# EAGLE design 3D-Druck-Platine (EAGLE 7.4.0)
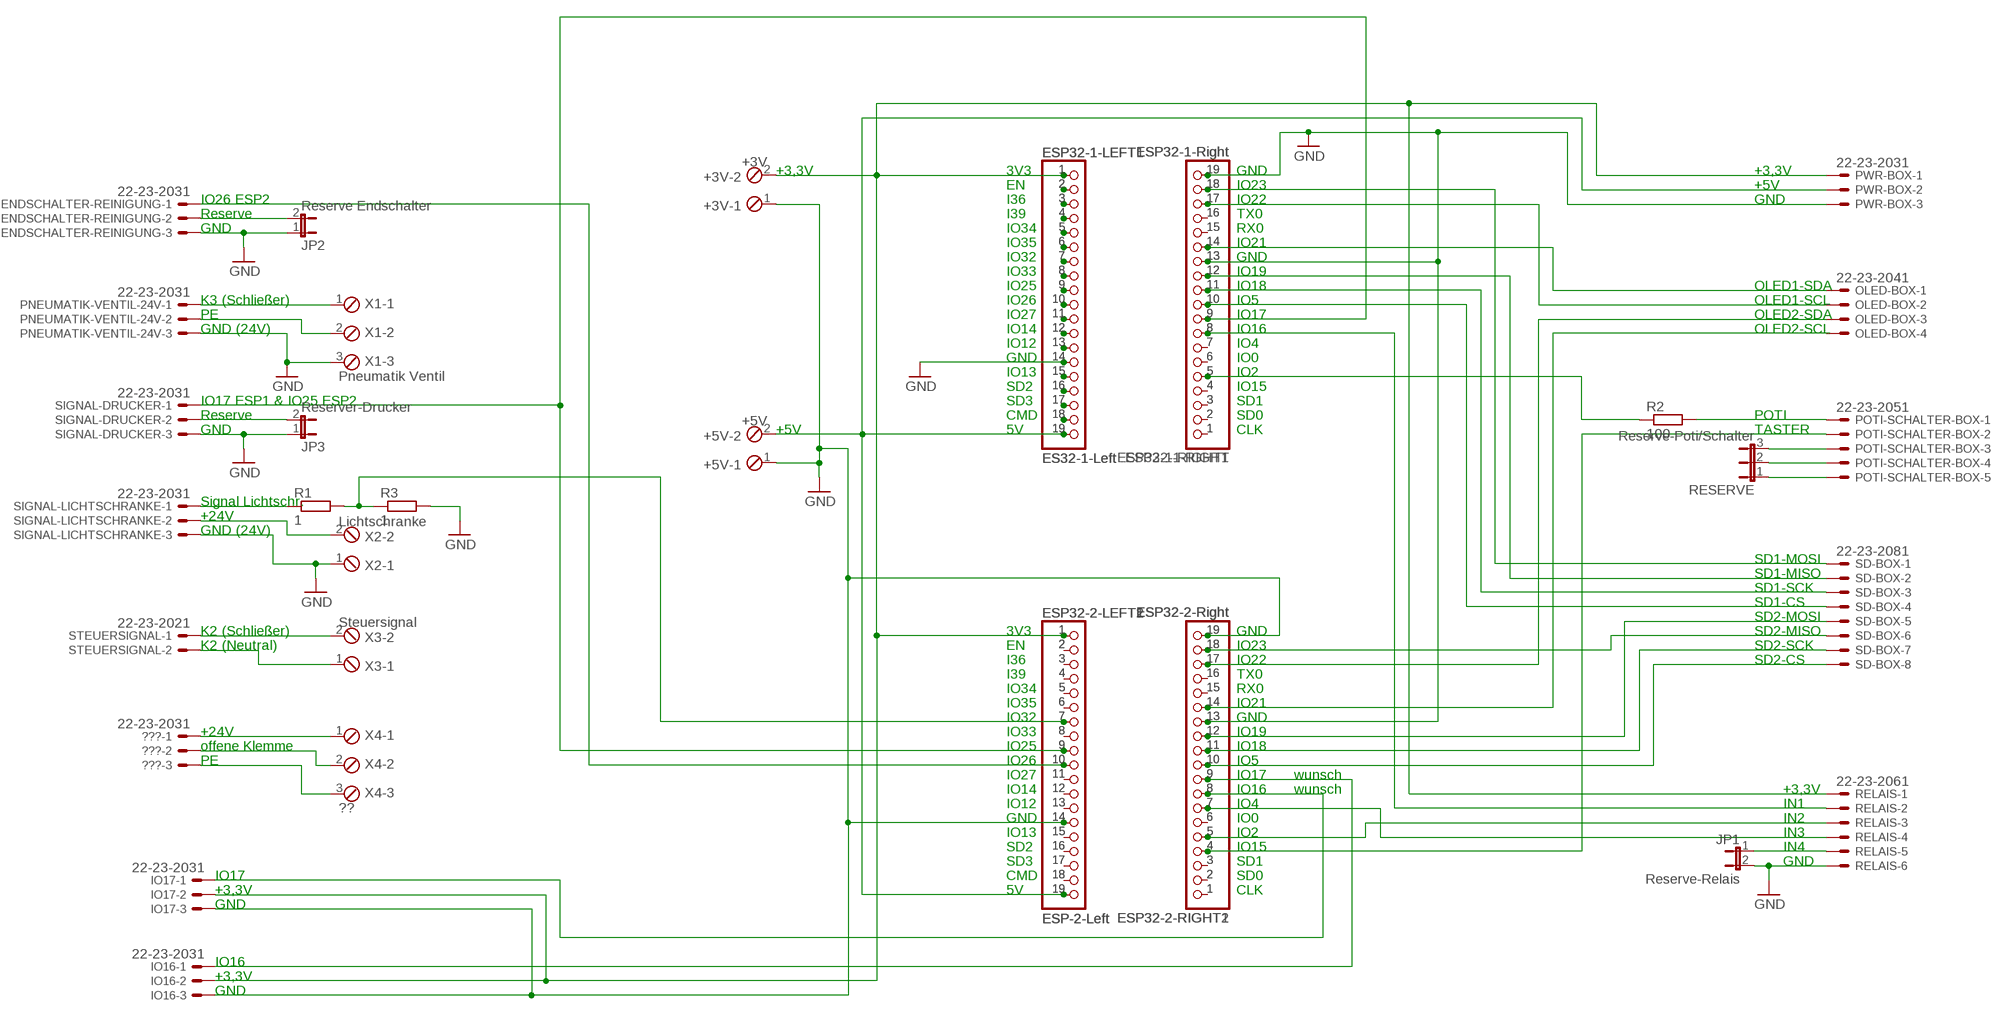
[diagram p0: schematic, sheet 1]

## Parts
+3V  +3V  MPT2  [2POL254]
+5V  +5V  MPT2  [2POL254]
???  22-23-2031  [22-23-2031]
ENDSCHALTER-REINIGUNG  22-23-2031  [22-23-2031]
ESP32-1-LEFT  ES32-1-Left  PINHD-1X19  [1X19]
ESP32-1-LEFT1  ES32-1-Left  PINHD-1X19  [1X19]
ESP32-1-RIGHT  ESP32-1-Right  PINHD-1X19  [1X19]
ESP32-1-RIGHT1  ESP32-1-Right  PINHD-1X19  [1X19]
ESP32-2-LEFT1  ESP-2-Left  PINHD-1X19  [1X19]
ESP32-2-LEFT2  ESP-2-Left  PINHD-1X19  [1X19]
ESP32-2-RIGHT1  ESP32-2-Right  PINHD-1X19  [1X19]
ESP32-2-RIGHT2  ESP32-2-Right  PINHD-1X19  [1X19]
IO16  22-23-2031  [22-23-2031]
IO17  22-23-2031  [22-23-2031]
JP1  Reserve-Relais  JP1E  [JP1]
JP2  Reserve Endschalter  JP1E  [JP1]
JP3  Reserver-Drucker  JP1E  [JP1]
OLED-BOX  22-23-2041  [22-23-2041]
PNEUMATIK-VENTIL-24V  22-23-2031  [22-23-2031]
POTI-SCHALTER-BOX  22-23-2051  [22-23-2051]
PWR-BOX  22-23-2031  [22-23-2031]
R1  1  R-EU_0207/10  [0207/10]
R2  100  R-EU_0207/10  [0207/10]
R3  1  R-EU_0207/10  [0207/10]
RELAIS  22-23-2061  [22-23-2061]
RESERVE  Reserve-Poti/Schalter  JP2E  [JP2]
SD-BOX  22-23-2081  [22-23-2081]
SIGNAL-DRUCKER  22-23-2031  [22-23-2031]
SIGNAL-LICHTSCHRANKE  22-23-2031  [22-23-2031]
STEUERSIGNAL  22-23-2021  [22-23-2021]
X1  Pneumatik Ventil  MPT3  [3POL254]
X2  Lichtschranke  MPT2  [2POL254]
X3  Steuersignal  MPT2  [2POL254]
X4  ??  MPT3  [3POL254]

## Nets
GND: +3V.1 +5V.1 ENDSCHALTER-REINIGUNG.3 ESP32-1-LEFT1.14 ESP32-1-LEFT.14 ESP32-1-RIGHT1.13 ESP32-1-RIGHT1.19 ESP32-1-RIGHT.13 ESP32-1-RIGHT.19 ESP32-2-LEFT1.14 ESP32-2-LEFT2.14 ESP32-2-RIGHT1.13 ESP32-2-RIGHT1.19 ESP32-2-RIGHT2.13 ESP32-2-RIGHT2.19 IO16.3 IO17.3 JP1.2 JP2.1 JP3.1 PNEUMATIK-VENTIL-24V.3 PWR-BOX.3 R3.2 RELAIS.6 SIGNAL-DRUCKER.3 SIGNAL-LICHTSCHRANKE.3 X1.3 X2.1
N$1: ESP32-1-LEFT1.2 ESP32-1-LEFT.2
N$2: POTI-SCHALTER-BOX.3 RESERVE.3
N$3: ESP32-1-LEFT1.3 ESP32-1-LEFT.3
N$3V: +3V.2 ESP32-1-LEFT1.1 ESP32-1-LEFT.1 ESP32-2-LEFT1.1 ESP32-2-LEFT2.1 IO16.2 IO17.2 PWR-BOX.1 RELAIS.1
N$4: POTI-SCHALTER-BOX.4 RESERVE.2
N$5: POTI-SCHALTER-BOX.5 RESERVE.1
N$5V: +5V.2 ESP32-1-LEFT1.19 ESP32-1-LEFT.19 ESP32-2-LEFT1.19 ESP32-2-LEFT2.19 PWR-BOX.2
N$6: ESP32-1-LEFT1.4 ESP32-1-LEFT.4
N$7: ESP32-1-LEFT1.5 ESP32-1-LEFT.5
N$8: ENDSCHALTER-REINIGUNG.2 JP2.2
N$9: ESP32-1-LEFT1.6 ESP32-1-LEFT.6
N$10: JP3.2 SIGNAL-DRUCKER.2
N$11: R1.1 SIGNAL-LICHTSCHRANKE.1
N$12: SIGNAL-LICHTSCHRANKE.2 X2.2
N$13: PNEUMATIK-VENTIL-24V.1 X1.1
N$14: STEUERSIGNAL.1 X3.2
N$15: STEUERSIGNAL.2 X3.1
N$16: PNEUMATIK-VENTIL-24V.2 X1.2
N$17: ???.1 X4.1
N$18: ???.2 X4.2
N$19: ???.3 X4.3
N$20: JP1.1 RELAIS.5
N$21: ESP32-1-LEFT1.7 ESP32-1-LEFT.7
N$22: ESP32-1-LEFT1.8 ESP32-1-LEFT.8
N$23: ESP32-1-LEFT1.9 ESP32-1-LEFT.9
N$24: ESP32-1-LEFT1.10 ESP32-1-LEFT.10
N$25: ESP32-1-LEFT1.11 ESP32-1-LEFT.11
N$26: ESP32-1-LEFT1.12 ESP32-1-LEFT.12
N$27: ESP32-1-LEFT1.13 ESP32-1-LEFT.13
N$28: ESP32-1-LEFT1.15 ESP32-1-LEFT.15
N$29: ESP32-1-LEFT1.16 ESP32-1-LEFT.16
N$30: ESP32-1-LEFT1.17 ESP32-1-LEFT.17
N$31: ESP32-1-LEFT1.18 ESP32-1-LEFT.18
N$32: ESP32-1-RIGHT1.1 ESP32-1-RIGHT.1
N$33: ESP32-1-RIGHT1.2 ESP32-1-RIGHT.2
N$34: ESP32-1-RIGHT1.3 ESP32-1-RIGHT.3
N$35: ESP32-1-RIGHT1.4 ESP32-1-RIGHT.4
N$37: ESP32-1-RIGHT1.7 ESP32-1-RIGHT.7
N$38: ESP32-1-RIGHT1.15 ESP32-1-RIGHT.15
N$39: ESP32-1-RIGHT1.16 ESP32-1-RIGHT.16
N$40: ESP32-2-LEFT1.2 ESP32-2-LEFT2.2
N$41: ESP32-2-LEFT1.3 ESP32-2-LEFT2.3
N$42: ESP32-2-LEFT1.4 ESP32-2-LEFT2.4
N$43: ESP32-2-LEFT1.5 ESP32-2-LEFT2.5
N$44: ESP32-2-LEFT1.6 ESP32-2-LEFT2.6
N$45: ESP32-2-LEFT1.8 ESP32-2-LEFT2.8
N$46: ESP32-2-LEFT1.11 ESP32-2-LEFT2.11
N$47: ESP32-2-LEFT1.12 ESP32-2-LEFT2.12
N$48: ESP32-2-LEFT1.13 ESP32-2-LEFT2.13
N$49: ESP32-2-LEFT1.15 ESP32-2-LEFT2.15
N$50: ESP32-2-LEFT1.16 ESP32-2-LEFT2.16
N$51: ESP32-2-LEFT1.17 ESP32-2-LEFT2.17
N$52: ESP32-2-LEFT1.18 ESP32-2-LEFT2.18
N$53: ESP32-2-RIGHT1.1 ESP32-2-RIGHT2.1
N$54: ESP32-2-RIGHT1.2 ESP32-2-RIGHT2.2
N$55: ESP32-2-RIGHT1.3 ESP32-2-RIGHT2.3
N$57: ESP32-2-RIGHT1.6 ESP32-2-RIGHT2.6
N$58: ESP32-2-RIGHT1.15 ESP32-2-RIGHT2.15
N$59: POTI-SCHALTER-BOX.1 R2.2
N$60: ESP32-1-RIGHT1.6 ESP32-1-RIGHT.6
N$101: ESP32-2-RIGHT1.16 ESP32-2-RIGHT2.16
N$ESP1-18: ESP32-1-RIGHT1.11 ESP32-1-RIGHT.11 SD-BOX.3
N$ESP1-IO2: ESP32-1-RIGHT1.5 ESP32-1-RIGHT.5 R2.1
N$ESP1-IO5: ESP32-1-RIGHT1.10 ESP32-1-RIGHT.10 SD-BOX.4
N$ESP1-IO16: ESP32-1-RIGHT1.8 ESP32-1-RIGHT.8 RELAIS.2
N$ESP1-IO17_ESP2-IO25: ESP32-1-RIGHT1.9 ESP32-1-RIGHT.9 ESP32-2-LEFT1.9 ESP32-2-LEFT2.9 SIGNAL-DRUCKER.1
N$ESP1-IO19: ESP32-1-RIGHT1.12 ESP32-1-RIGHT.12 SD-BOX.2
N$ESP1-IO21: ESP32-1-RIGHT1.14 ESP32-1-RIGHT.14 OLED-BOX.1
N$ESP1-IO22: ESP32-1-RIGHT1.17 ESP32-1-RIGHT.17 OLED-BOX.2
N$ESP1-IO23: ESP32-1-RIGHT1.18 ESP32-1-RIGHT.18 SD-BOX.1
N$ESP2-IO2: ESP32-2-RIGHT1.5 ESP32-2-RIGHT2.5 RELAIS.3
N$ESP2-IO4: ESP32-2-RIGHT1.7 ESP32-2-RIGHT2.7 RELAIS.4
N$ESP2-IO5: ESP32-2-RIGHT1.10 ESP32-2-RIGHT2.10 SD-BOX.8
N$ESP2-IO15: ESP32-2-RIGHT1.4 ESP32-2-RIGHT2.4 POTI-SCHALTER-BOX.2
N$ESP2-IO16: ESP32-2-RIGHT1.8 ESP32-2-RIGHT2.8 IO17.1
N$ESP2-IO17: ESP32-2-RIGHT1.9 ESP32-2-RIGHT2.9 IO16.1
N$ESP2-IO18: ESP32-2-RIGHT1.11 ESP32-2-RIGHT2.11 SD-BOX.7
N$ESP2-IO19: ESP32-2-RIGHT1.12 ESP32-2-RIGHT2.12 SD-BOX.5
N$ESP2-IO21: ESP32-2-RIGHT1.14 ESP32-2-RIGHT2.14 OLED-BOX.4
N$ESP2-IO22: ESP32-2-RIGHT1.17 ESP32-2-RIGHT2.17 OLED-BOX.3
N$ESP2-IO23: ESP32-2-RIGHT1.18 ESP32-2-RIGHT2.18 SD-BOX.6
N$ESP2-IO26: ENDSCHALTER-REINIGUNG.1 ESP32-2-LEFT1.10 ESP32-2-LEFT2.10
N$ESP2-IO32: ESP32-2-LEFT1.7 ESP32-2-LEFT2.7 R1.2 R3.1

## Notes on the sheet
- +3,3V | 3V3 | GND | +3,3V
- EN | IO23 | +5V
- IO26 ESP2 | I36 | IO22 | GND
- Reserve | I39 | TX0
- GND | IO34 | RX0
- IO35 | IO21
- IO32 | GND
- IO33 | IO19
- IO25 | IO18 | OLED1-SDA
- K3 (Schließer) | IO26 | IO5 | OLED1-SCL
- PE | IO27 | IO17 | OLED2-SDA
- GND (24V) | IO14 | IO16 | OLED2-SCL
- IO12 | IO4
- GND | IO0
- IO13 | IO2
- SD2 | IO15
- IO17 ESP1 & IO25 ESP2 | SD3 | SD1
- Reserve | CMD | SD0 | POTI
- GND | +5V | 5V | CLK | TASTER
- Signal Lichtschr.
- +24V
- GND (24V)
- SD1-MOSI
- SD1-MISO
- SD1-SCK
- SD1-CS
- SD2-MOSI
- K2 (Schließer) | 3V3 | GND | SD2-MISO
- K2 (Neutral) | EN | IO23 | SD2-SCK
- I36 | IO22 | SD2-CS
- I39 | TX0
- IO34 | RX0
- IO35 | IO21
- IO32 | GND
- +24V | IO33 | IO19
- offene Klemme | IO25 | IO18
- PE | IO26 | IO5
- IO27 | IO17 | wunsch
- IO14 | IO16 | wunsch | +3,3V
- IO12 | IO4 | IN1
- GND | IO0 | IN2
- IO13 | IO2 | IN3
- SD2 | IO15 | IN4
- SD3 | SD1 | GND
- IO17 | CMD | SD0
- +3,3V | 5V | CLK
- GND
- IO16
- +3,3V
- GND

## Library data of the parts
+3V +5V X2 X3 = con-phoenix-254:MPT2: PHOENIX CONNECTOR; OC_FARNELL: unknown; OC_NEWARK: unknown
??? ENDSCHALTER-REINIGUNG IO16 IO17 PNEUMATIK-VENTIL-24V PWR-BOX SIGNAL-DRUCKER SIGNAL-LICHTSCHRANKE = con-molex:22-23-2031: .100" (2.54mm) Center Header - 3 Pin; MF: MOLEX; MPN: 22-23-2031; OC_FARNELL: 1462950; OC_NEWARK: 30C0862
ESP32-1-LEFT ESP32-1-LEFT1 ESP32-1-RIGHT ESP32-1-RIGHT1 ESP32-2-LEFT1 ESP32-2-LEFT2 ESP32-2-RIGHT1 ESP32-2-RIGHT2 = pinhead:PINHD-1X19: PIN HEADER
JP1-JP3 = jumper:JP1E: JUMPER
OLED-BOX = con-molex:22-23-2041: .100" (2.54mm) Center Header - 4 Pin; MF: MOLEX; MPN: 22-23-2041; OC_FARNELL: 1462920; OC_NEWARK: 38C0355
POTI-SCHALTER-BOX = con-molex:22-23-2051: .100" (2.54mm) Center Header - 5 Pin; MF: MOLEX; MPN: 22-23-2051; OC_FARNELL: 1462952; OC_NEWARK: 38C9178
R1-R3 = rcl:R-EU_: RESISTOR, European symbol
RELAIS = con-molex:22-23-2061: .100" (2.54mm) Center Header - 6 Pin; MF: MOLEX; MPN: 22-23-2061; OC_FARNELL: 1462922; OC_NEWARK: 27C1933
RESERVE = jumper:JP2E: JUMPER
SD-BOX = con-molex:22-23-2081: .100" (2.54mm) Center Header - 8 Pin; MF: MOLEX; MPN: 22-23-2081; OC_FARNELL: 1756826; OC_NEWARK: 01C7592
STEUERSIGNAL = con-molex:22-23-2021: .100" (2.54mm) Center Header - 2 Pin; MF: MOLEX; MPN: 22-23-2021; OC_FARNELL: 1462926; OC_NEWARK: 25C3832
X1 X4 = con-phoenix-254:MPT3: PHOENIX CONNECTOR; OC_FARNELL: unknown; OC_NEWARK: unknown

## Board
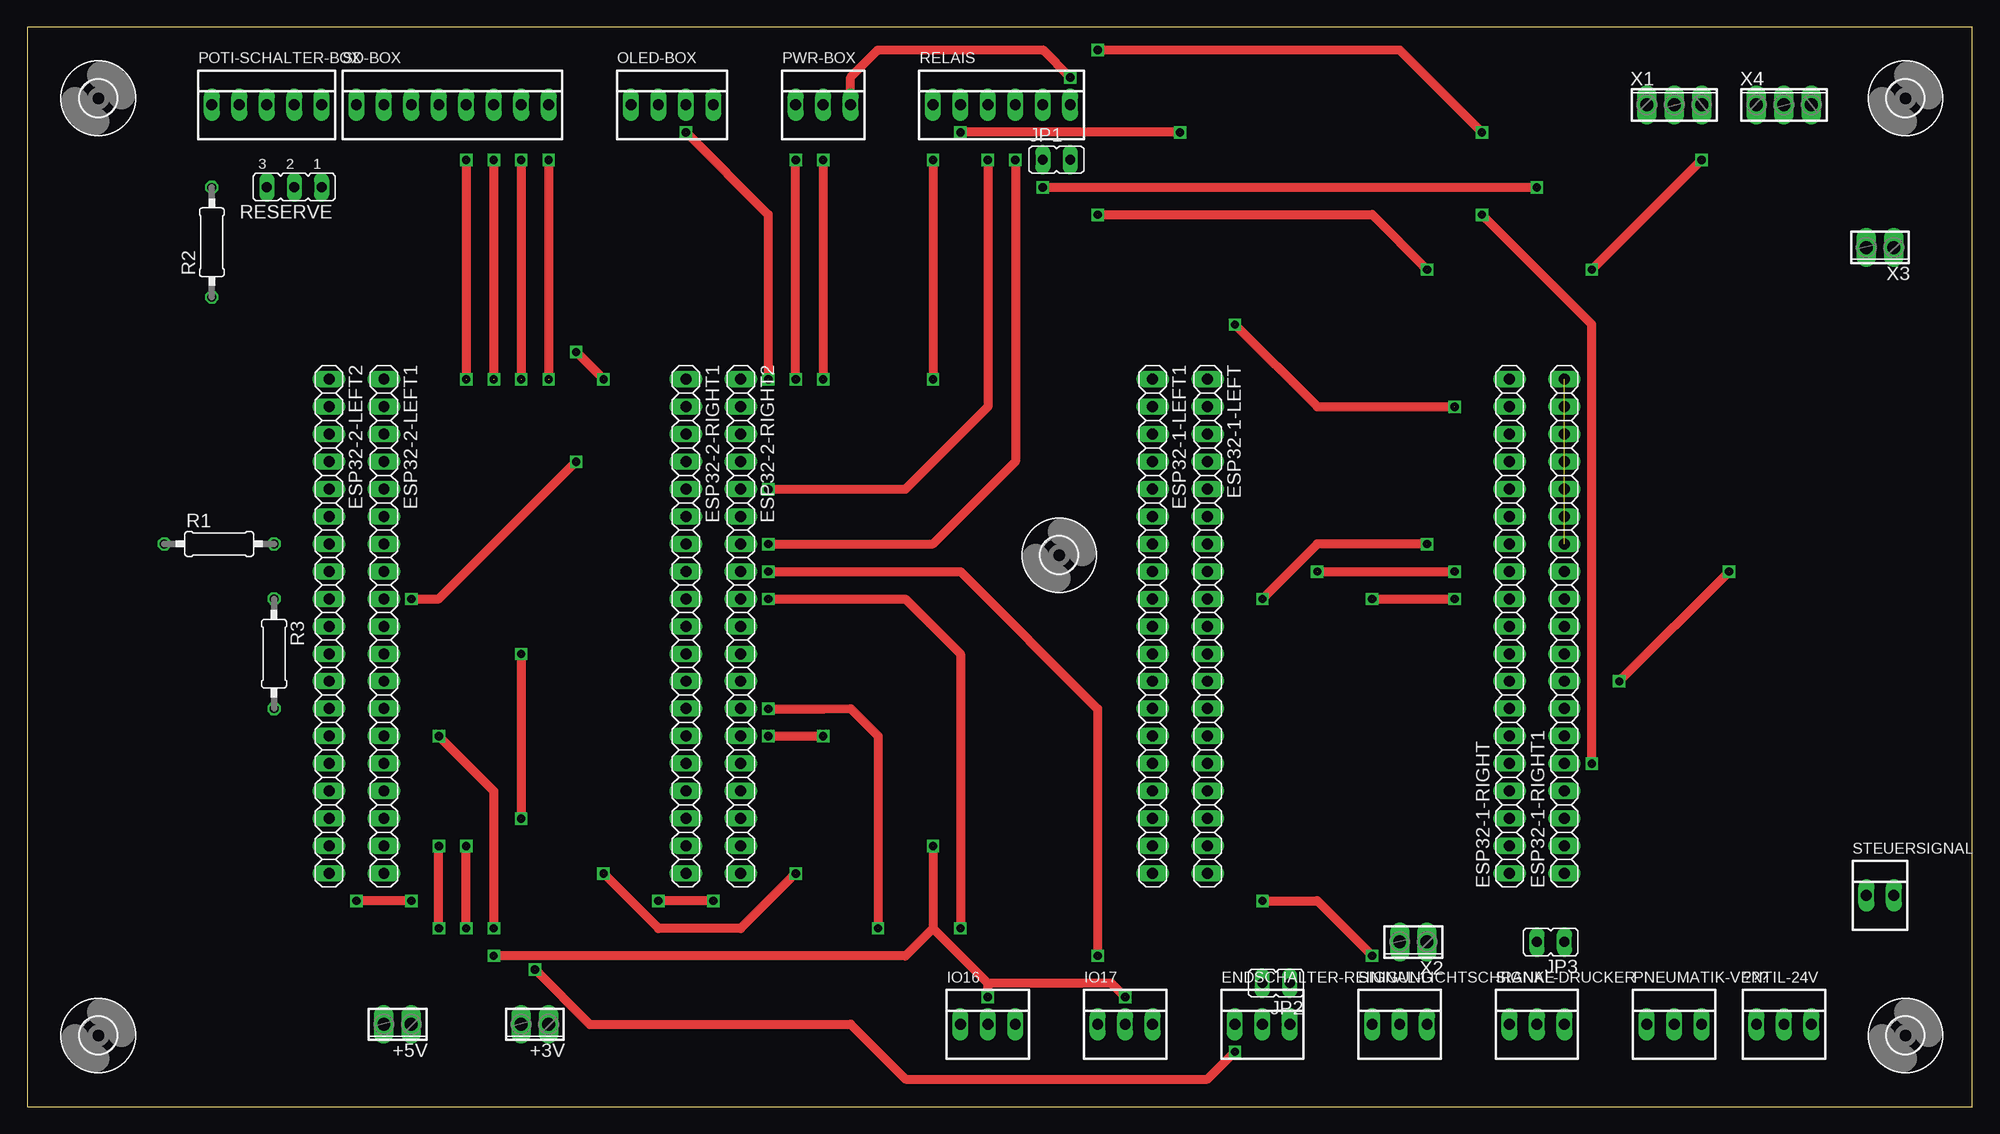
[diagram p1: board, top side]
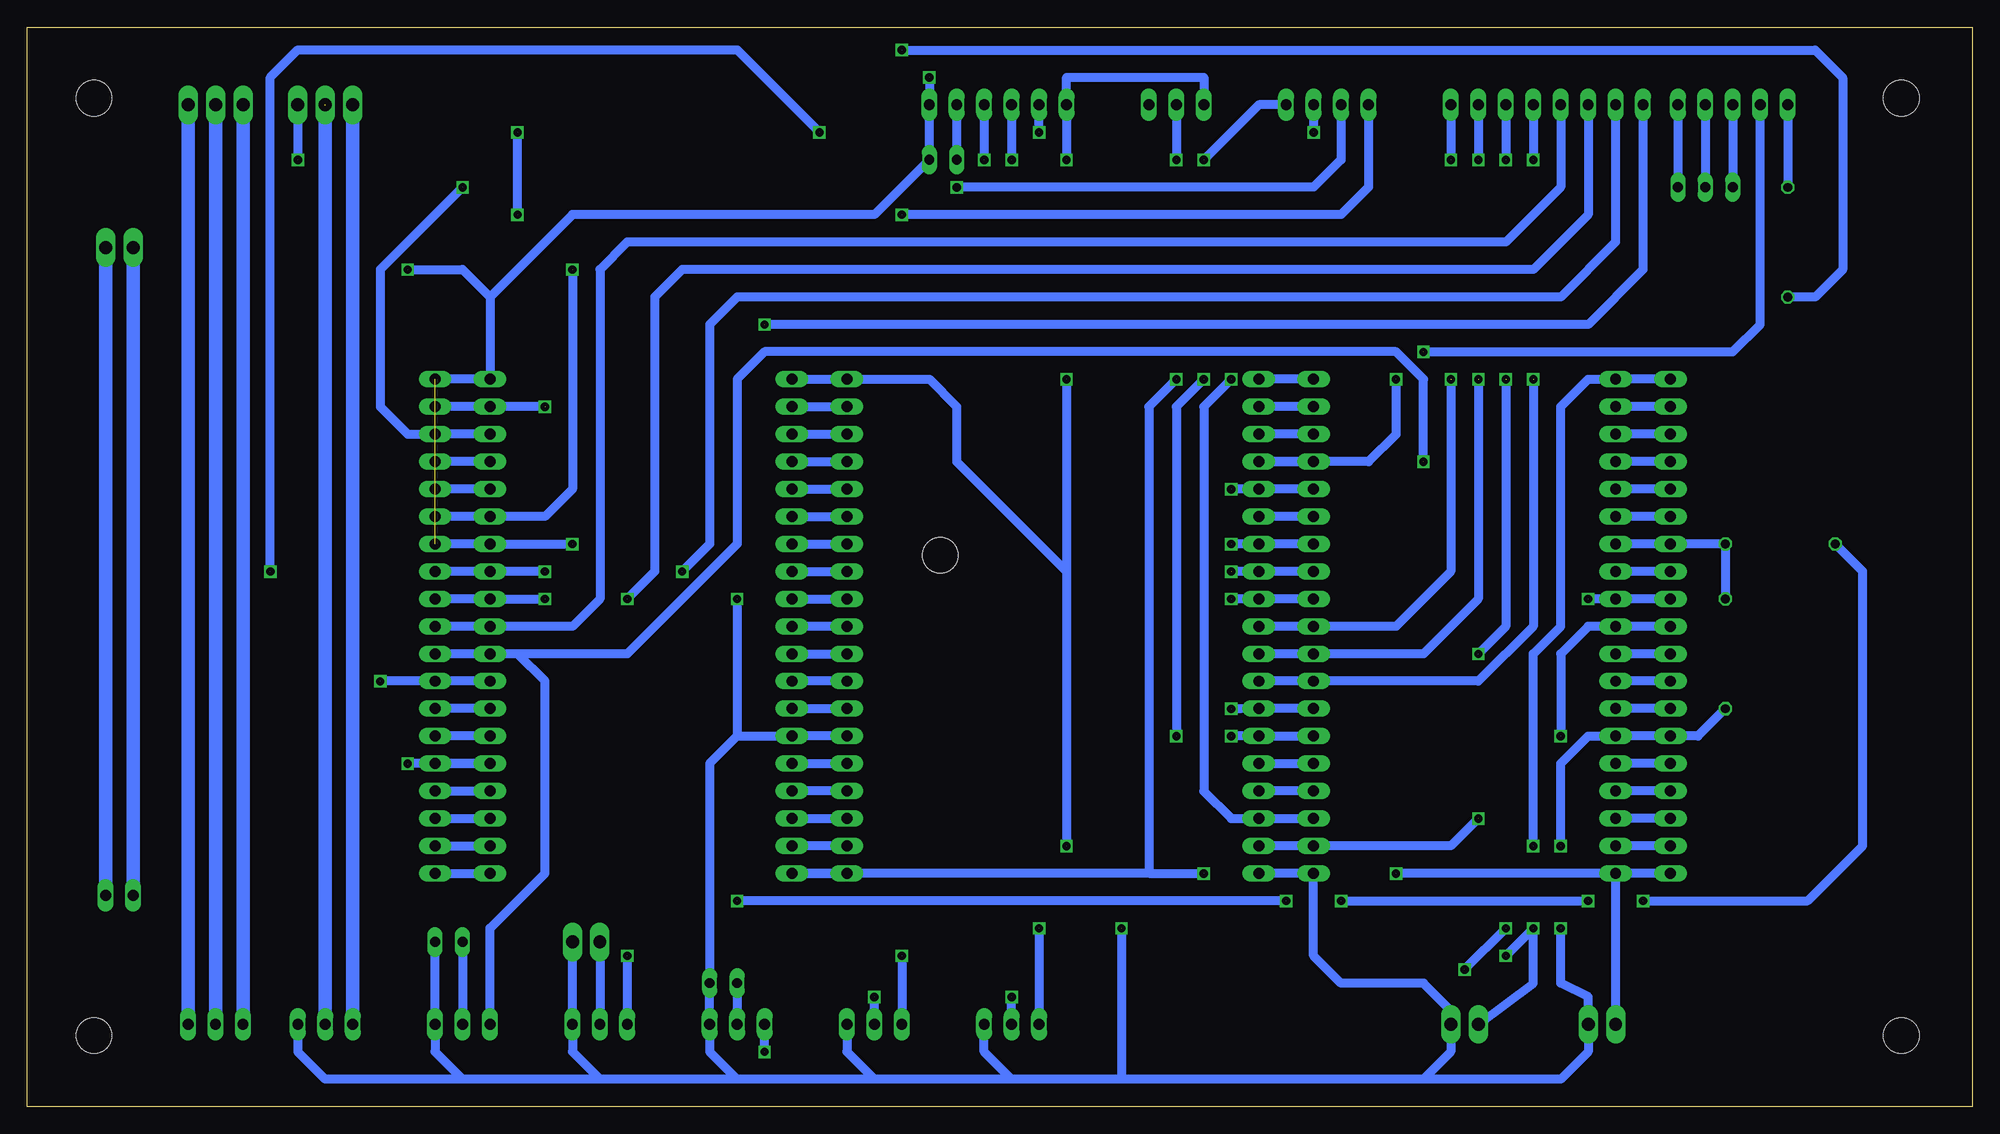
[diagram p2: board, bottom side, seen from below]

Size 180 x 99.92 mm. Coordinates in mm from the lower left corner, seen from the top.
Outline: 0,0 180,0 180,99.92 0,99.92 0,0
Copper layers 16: Bottom 0.035mm
Design rules "Multi-CB_1L_100µm-Tracks_OL35µm": minimum track width 0.1mm, minimum drill 0.2mm, track to track 0.1mm, track to pad 0.1mm, pad to pad 0.1mm, via to via 0.1mm, smd to smd 0mil, copper to edge 0.2mm, drill to drill 0.2mm, minimum pad ring 0.125mm, minimum via ring 0.1mm, stop-mask expansion 2mil, vias tented up to drill 0.45mm, thermal gap 0.2mm

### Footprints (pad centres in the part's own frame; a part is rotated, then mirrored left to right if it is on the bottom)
2POL254 = drill 1.2 long: 1 -1.27,0; 2 1.27,0
22-23-2031 = drill 1 long: 1 -2.54,0; 2 0,0; 3 2.54,0
1X19 = drill 1.016 long: 1 -22.86,0; 2 -20.32,0; 3 -17.78,0; 4 -15.24,0; 5 -12.7,0; 6 -10.16,0; 7 -7.62,0; 8 -5.08,0; 9 -2.54,0; 10 0,0; 11 2.54,0; 12 5.08,0; 13 7.62,0; 14 10.16,0; 15 12.7,0; 16 15.24,0; 17 17.78,0; 18 20.32,0; 19 22.86,0
JP1 = drill 0.914 long: 1 0,-1.27; 2 0,1.27
22-23-2041 = drill 1 long: 1 -3.81,0; 2 -1.27,0; 3 1.27,0; 4 3.81,0
22-23-2051 = drill 1 long: 1 -5.08,0; 2 -2.54,0; 3 0,0; 4 2.54,0; 5 5.08,0
0207/10 = drill 0.813 octagon: 1 -5.08,0; 2 5.08,0
22-23-2061 = drill 1 long: 1 -6.35,0; 2 -3.81,0; 3 -1.27,0; 4 1.27,0; 5 3.81,0; 6 6.35,0
JP2 = drill 0.914 long: 1 -2.54,0; 2 0,0; 3 2.54,0
22-23-2081 = drill 1 long: 1 -8.89,0; 2 -6.35,0; 3 -3.81,0; 4 -1.27,0; 5 1.27,0; 6 3.81,0; 7 6.35,0; 8 8.89,0
22-23-2021 = drill 1 long: 1 -1.27,0; 2 1.27,0
3,3 = hole 3.3: 0,0
3POL254 = drill 1.2 long: 1 -2.54,0; 2 0,0; 3 2.54,0

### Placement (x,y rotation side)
+3V  46.99,7.64 180 top
+5V  34.29,7.64 180 top
???  162.56,7.64 0 top
ENDSCHALTER-REINIGUNG  114.3,7.64 0 top
ESP32-1-LEFT  109.22,44.47 270 top
ESP32-1-LEFT1  104.14,44.47 270 top
ESP32-1-RIGHT  137.16,44.47 90 top
ESP32-1-RIGHT1  142.24,44.47 90 top
ESP32-2-LEFT1  33.02,44.47 270 top
ESP32-2-LEFT2  27.94,44.47 270 top
ESP32-2-RIGHT1  60.96,44.47 270 top
ESP32-2-RIGHT2  66.04,44.47 270 top
IO16  88.9,7.64 0 top
IO17  101.6,7.64 0 top
JP1  95.25,87.65 270 top
JP2  115.57,11.45 90 top
JP3  140.97,15.26 90 top
OLED-BOX  59.69,92.73 0 top
PNEUMATIK-VENTIL-24V  152.4,7.64 0 top
POTI-SCHALTER-BOX  22.18,92.73 0 top
PWR-BOX  73.66,92.73 0 top
R1  17.78,52.09 0 top
R2  17.1,80.01 90 top
R3  22.86,41.93 270 top
RELAIS  90.17,92.73 0 top
RESERVE  24.72,85.11 180 top
SD-BOX  39.37,92.73 0 top
SIGNAL-DRUCKER  139.7,7.64 0 top
SIGNAL-LICHTSCHRANKE  127,7.64 0 top
STEUERSIGNAL  171.45,19.57 0 top
U$1  [3,3]  6.6,6.6 0 top
U$2  [3,3]  6.6,93.33 0 top
U$3  [3,3]  173.8,93.33 0 top
U$4  [3,3]  173.8,6.6 0 top
U$5  [3,3]  95.5,51.05 0 top
X1  152.4,92.73 0 top
X2  128.27,15.26 180 top
X3  171.45,79.53 180 top
X4  162.56,92.73 0 top

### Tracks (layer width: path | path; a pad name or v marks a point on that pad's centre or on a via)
GND  (14 unrouted)
  Top 0.813: 154.94,87.65 144.78,77.49 | 38.1,16.53 38.1,24.15 | 78.74,16.53 78.74,34.31 76.2,36.85 arc-2 68.58,36.83 | PWR-BOX.3 76.2,95.27 78.74,97.81 93.98,97.81 96.52,95.27 | 129.54,52.09 119.38,52.09 114.3,47.01
  Bottom 0.813: 137.16,74.95 ESP32-1-RIGHT.19 ESP32-1-RIGHT1.19 | JP3.1 SIGNAL-DRUCKER.3 142.24,5.1 139.7,2.56 | X1.3 154.94,87.65 | PNEUMATIK-VENTIL-24V.3 154.94,5.1 152.4,2.56 139.7,2.56 | X2.1 SIGNAL-LICHTSCHRANKE.3 129.54,5.1 127,2.56 | 50.8,2.56 48.26,5.1 +3V.1 48.26,8.89 50.8,11.43 50.8,11.45 58.42,11.45 60.96,13.99 ESP32-2-RIGHT1.19 ESP32-2-RIGHT2.19 | 50.8,2.56 78.74,2.56 | 88.9,2.56 101.6,2.56 | 101.6,2.56 114.3,2.56 | 114.3,2.56 127,2.56 | 127,2.56 139.7,2.56 | 50.8,2.56 38.1,2.56 35.56,5.1 +5V.1 35.56,10.18 38.1,11.45 38.1,16.53 | 114.3,34.31 116.84,31.77 JP2.1 ENDSCHALTER-REINIGUNG.3 116.84,5.1 114.3,2.56 | 114.3,34.31 ESP32-1-LEFT.14 ESP32-1-LEFT1.14 | R3.2 25.4,34.31 ESP32-2-LEFT2.14 ESP32-2-LEFT1.14 35.56,34.31 38.1,31.77 38.1,24.15 | 78.74,16.53 78.74,2.56 | 96.52,95.27 RELAIS.6 JP1.2 101.6,82.57 129.54,82.57 137.16,74.95 | 144.78,77.49 139.7,77.49 137.16,74.95 | IO17.3 104.14,5.1 101.6,2.56 | 78.74,2.56 88.9,2.56 | 88.9,2.56 91.44,5.1 IO16.3 | ESP32-1-RIGHT1.13 ESP32-1-RIGHT.13 129.54,52.09 | 114.3,47.01 114.3,34.31 | ESP32-2-RIGHT1.13 ESP32-2-RIGHT2.13 arc-1 68.58,36.83
N$1
  Bottom 0.813: ESP32-1-LEFT.2 ESP32-1-LEFT1.2
N$2
  Bottom 0.813: POTI-SCHALTER-BOX.3 RESERVE.3
N$3
  Bottom 0.813: ESP32-1-LEFT.3 ESP32-1-LEFT1.3 104.14,62.23
N$3V  (13 unrouted)
  Top 0.813: 83.82,87.65 83.82,67.33 | 40.64,16.53 40.64,24.15 | 83.82,24.15 83.82,16.53 | 88.9,10.16 88.9,11.43 | 88.9,11.43 88.9,11.45 83.82,16.53 | 101.6,10.18 101.58,10.18 100.33,11.43 88.9,11.43 | 83.82,16.53 83.82,16.51 81.28,13.97 43.2,13.97 43.18,13.99
  Bottom 0.813: PWR-BOX.1 71.12,95.27 83.82,95.27 RELAIS.1 83.82,87.65 | +3V.2 40.64,11.45 40.64,16.53 43.18,13.99 | 40.64,24.15 40.64,41.93 38.1,44.47 38.1,64.79 35.56,67.33 ESP32-2-LEFT1.1 ESP32-2-LEFT2.1 | 83.82,49.55 93.98,59.71 93.98,64.79 96.52,67.33 ESP32-1-LEFT1.1 ESP32-1-LEFT.1 | 83.82,49.55 83.82,24.15 | 83.82,67.33 83.82,49.55 | IO16.2 88.9,10.18 | IO17.2 101.6,10.18
N$4
  Bottom 0.813: POTI-SCHALTER-BOX.4 RESERVE.2
N$5
  Bottom 0.813: POTI-SCHALTER-BOX.5 RESERVE.1
N$5V  (6 unrouted)
  Top 0.813: 73.66,87.65 73.66,67.33 | 53.34,21.61 58.42,16.53 58.42,16.51 66.04,16.51 71.12,21.59
  Bottom 0.813: PWR-BOX.2 73.66,87.65 | 76.2,21.61 ESP32-1-LEFT.19 ESP32-1-LEFT1.19 104.14,21.59 | ESP32-2-LEFT1.19 +5V.2 | ESP32-2-LEFT1.19 53.34,21.61 | 73.66,67.33 76.2,64.79 76.2,21.61 | ESP32-2-LEFT2.19 ESP32-2-LEFT1.19 | 76.2,21.61 71.14,21.61 71.12,21.59
N$6
  Bottom 0.813: ESP32-1-LEFT.4 ESP32-1-LEFT1.4 104.14,59.69
N$7
  Bottom 0.813: ESP32-1-LEFT.5 ESP32-1-LEFT1.5
N$8
  Bottom 0.813: JP2.2 ENDSCHALTER-REINIGUNG.2
N$9
  Bottom 0.813: ESP32-1-LEFT.6 ESP32-1-LEFT1.6
N$10
  Bottom 0.813: JP3.2 SIGNAL-DRUCKER.2
N$11  (6 unrouted)
  Top 0.813: 63.5,19.07 58.42,19.07 | 35.56,19.07 30.48,19.07 | 114.3,19.07 119.38,19.07 124.46,13.99
  Bottom 0.813: 58.42,19.07 35.56,19.07 | 30.48,19.07 15.24,19.07 10.16,24.15 10.16,49.55 R1.1 | 63.5,19.07 114.3,19.07 | 124.46,13.99 SIGNAL-LICHTSCHRANKE.1
N$12
  Bottom 0.813: X2.2 SIGNAL-LICHTSCHRANKE.2
N$13
  Bottom 1.27: X1.1 PNEUMATIK-VENTIL-24V.1
N$14
  Bottom 1.27: X3.2 STEUERSIGNAL.1
N$15
  Bottom 1.27: X3.1 STEUERSIGNAL.2
N$16  (1 unrouted)
  Bottom 1.27: PNEUMATIK-VENTIL-24V.2 152.4,92.71
N$17
  Bottom 1.27: X4.1 ???.1
N$18
  Bottom 1.27: ???.2 X4.2
N$19
  Bottom 1.27: X4.3 ???.3
N$20
  Bottom 0.813: RELAIS.5 JP1.1
N$21
  Bottom 0.813: ESP32-1-LEFT.7 ESP32-1-LEFT1.7
N$22
  Bottom 0.813: ESP32-1-LEFT.8 ESP32-1-LEFT1.8 104.14,49.53
N$23
  Bottom 0.813: ESP32-1-LEFT.9 ESP32-1-LEFT1.9
N$24
  Bottom 0.813: ESP32-1-LEFT1.10 ESP32-1-LEFT.10
N$25
  Bottom 0.813: ESP32-1-LEFT.11 ESP32-1-LEFT1.11 104.14,41.91
N$26
  Bottom 0.813: ESP32-1-LEFT1.12 ESP32-1-LEFT.12
N$27
  Bottom 0.813: ESP32-1-LEFT.13 ESP32-1-LEFT1.13
N$28
  Bottom 0.813: ESP32-1-LEFT.15 ESP32-1-LEFT1.15 104.14,31.75
N$29
  Bottom 0.813: ESP32-1-LEFT1.16 ESP32-1-LEFT.16
N$30
  Bottom 0.813: ESP32-1-LEFT.17 ESP32-1-LEFT1.17 104.14,26.67
N$31
  Bottom 0.813: ESP32-1-LEFT1.18 ESP32-1-LEFT.18
N$32
  Bottom 0.813: ESP32-1-RIGHT1.1 ESP32-1-RIGHT.1
N$33
  Bottom 0.813: ESP32-1-RIGHT1.2 ESP32-1-RIGHT.2
N$34
  Bottom 0.813: ESP32-1-RIGHT1.3 ESP32-1-RIGHT.3
N$35
  Bottom 0.813: ESP32-1-RIGHT1.4 ESP32-1-RIGHT.4
N$37
  Bottom 0.813: ESP32-1-RIGHT.7 ESP32-1-RIGHT1.7
N$38
  Bottom 0.813: ESP32-1-RIGHT.15 ESP32-1-RIGHT1.15
N$39
  Bottom 0.813: ESP32-1-RIGHT.16 ESP32-1-RIGHT1.16
N$40
  Bottom 0.813: ESP32-2-LEFT2.2 ESP32-2-LEFT1.2
N$41
  Bottom 0.813: ESP32-2-LEFT2.3 ESP32-2-LEFT1.3
N$42
  Bottom 0.813: ESP32-2-LEFT2.4 ESP32-2-LEFT1.4
N$43
  Bottom 0.813: ESP32-2-LEFT2.5 ESP32-2-LEFT1.5
N$44
  Bottom 0.813: ESP32-2-LEFT2.6 ESP32-2-LEFT1.6
N$45
  Bottom 0.813: ESP32-2-LEFT2.8 ESP32-2-LEFT1.8
N$46
  Bottom 0.813: ESP32-2-LEFT2.11 ESP32-2-LEFT1.11
N$47
  Bottom 0.813: ESP32-2-LEFT2.12 ESP32-2-LEFT1.12
N$48
  Bottom 0.813: ESP32-2-LEFT2.13 ESP32-2-LEFT1.13
N$49
  Bottom 0.813: ESP32-2-LEFT2.15 ESP32-2-LEFT1.15
N$50
  Bottom 0.813: ESP32-2-LEFT2.16 ESP32-2-LEFT1.16
N$51
  Bottom 0.813: ESP32-2-LEFT2.17 ESP32-2-LEFT1.17
N$52
  Bottom 0.813: ESP32-2-LEFT2.18 ESP32-2-LEFT1.18
N$53
  Bottom 0.813: ESP32-2-RIGHT1.1 ESP32-2-RIGHT2.1
N$54
  Bottom 0.813: ESP32-2-RIGHT1.2 ESP32-2-RIGHT2.2
N$55
  Bottom 0.813: ESP32-2-RIGHT1.3 ESP32-2-RIGHT2.3
N$57
  Bottom 0.813: ESP32-2-RIGHT1.6 ESP32-2-RIGHT2.6
N$58
  Bottom 0.813: ESP32-2-RIGHT2.15 ESP32-2-RIGHT1.15
N$59
  Bottom 0.813: POTI-SCHALTER-BOX.1 R2.2
N$60
  Bottom 0.813: ESP32-1-RIGHT.6 ESP32-1-RIGHT1.6
N$67  (via drill 0.76)
  other vias: 93.98,85.09
N$68  (1 unrouted)
N$74  (1 unrouted)
N$75  (1 unrouted)
N$76  (1 unrouted)
N$77  (1 unrouted)
N$78  (1 unrouted)
N$79  (1 unrouted)
N$100  (1 unrouted)
N$101
  Bottom 0.813: ESP32-2-RIGHT1.16 ESP32-2-RIGHT2.16
N$ESP1-18  (3 unrouted)
  Top 0.813: 124.46,47.01 132.08,47.01
  Bottom 0.813: SD-BOX.3 35.56,82.57 40.64,77.49 119.38,77.49 121.92,74.95 121.92,49.55 124.46,47.01 | ESP32-1-RIGHT1.11 ESP32-1-RIGHT.11 132.08,47.01
N$ESP1-IO2  (4 unrouted)
  Top 0.813: 144.78,31.75 144.78,72.39 134.62,82.55 | 134.62,90.17 127,97.79 99.06,97.79
  Bottom 0.813: 144.78,31.75 144.76,31.77 ESP32-1-RIGHT1.5 142.22,31.75 | 134.62,82.55 134.62,90.17 | 99.06,97.79 14.56,97.79 12.02,95.25 12.02,77.47 14.56,74.93 R2.1 | ESP32-1-RIGHT.5 142.22,31.77 142.24,31.75 142.22,31.75 | 137.16,31.75 142.22,31.75
N$ESP1-IO5
  Bottom 0.813: SD-BOX.4 38.1,85.11 43.18,80.03 124.46,80.03 127,77.49 127,47.01 129.54,44.47 ESP32-1-RIGHT.10 ESP32-1-RIGHT1.10
N$ESP1-IO16  (4 unrouted)
  Top 0.813: 147.32,39.39 157.48,49.55 | 106.68,90.19 86.36,90.19
  Bottom 0.813: ESP32-1-RIGHT1.8 ESP32-1-RIGHT.8 147.32,39.39 | 157.48,49.55 157.48,95.27 154.94,97.81 114.3,97.81 106.68,90.19 | 86.36,90.19 RELAIS.2
N$ESP1-IO17_ESP2-IO25  (2 unrouted)
  Top 0.813: 35.56,47.01 38.1,47.01 50.8,59.71
  Bottom 0.813: 134.62,41.93 124.46,41.93 114.3,52.09 114.3,67.33 111.76,69.87 53.34,69.87 50.8,67.33 50.8,59.71 | 134.62,41.93 ESP32-1-RIGHT.9 ESP32-1-RIGHT1.9 | 35.56,47.01 ESP32-2-LEFT1.9 ESP32-2-LEFT2.9 | SIGNAL-DRUCKER.1 137.16,16.53 132.08,21.61 132.08,39.39 134.62,41.93
N$ESP1-IO19  (2 unrouted)
  Top 0.813: 119.38,49.55 132.08,49.55
  Bottom 0.813: SD-BOX.2 33.02,80.03 38.1,74.95 114.3,74.95 116.84,72.41 116.84,52.09 119.38,49.55 | 132.08,49.55 ESP32-1-RIGHT.12 ESP32-1-RIGHT1.12
N$ESP1-IO21  (4 unrouted)
  Top 0.813: 99.06,82.57 124.46,82.57 129.54,77.49
  Bottom 0.813: OLED-BOX.1 55.88,85.11 58.42,82.57 99.06,82.57 | 129.54,77.49 129.54,57.17 132.08,54.63 ESP32-1-RIGHT.14 ESP32-1-RIGHT1.14
N$ESP1-IO22  (via drill 0.6)  (1 unrouted)
  Top 0.813: v93.98,85.11 139.7,85.11
  Bottom 0.813: OLED-BOX.2 58.42,87.65 60.96,85.11 v93.98,85.11 | ESP32-1-RIGHT.17 ESP32-1-RIGHT1.17 144.78,62.25 147.32,64.79 147.32,77.49 139.7,85.11
N$ESP1-IO23  (2 unrouted)
  Top 0.813: 111.76,72.41 119.38,64.79 132.08,64.79
  Bottom 0.813: SD-BOX.1 30.48,77.49 35.56,72.41 111.76,72.41 | 132.08,64.79 ESP32-1-RIGHT.18 ESP32-1-RIGHT1.18
N$ESP2-IO2  (4 unrouted)
  Top 0.813: 68.58,57.17 81.28,57.17 88.9,64.79 88.9,87.65
  Bottom 0.813: ESP32-2-RIGHT1.5 ESP32-2-RIGHT2.5 68.58,57.17 | RELAIS.3 88.9,87.65
N$ESP2-IO4  (4 unrouted)
  Top 0.813: 68.58,52.09 83.82,52.09 91.44,59.71 91.44,87.65
  Bottom 0.813: ESP32-2-RIGHT1.7 ESP32-2-RIGHT2.7 68.58,52.09 | RELAIS.4 91.44,87.65
N$ESP2-IO5  (via drill 0.76)  (4 unrouted)
  Top 0.813: 48.26,87.65 v48.26,87.63 48.26,67.33
  Bottom 0.813: SD-BOX.8 48.26,87.65 | 48.26,67.33 48.26,49.55 53.34,44.47 ESP32-2-RIGHT1.10 ESP32-2-RIGHT2.10
N$ESP2-IO15  (via drill 0.76)  (2 unrouted)
  Top 0.813: 53.34,67.33 50.8,69.87
  Bottom 0.813: 53.34,67.33 v53.34,67.31 53.34,62.23 55.88,59.69 60.96,59.69 | 50.8,69.87 22.18,69.87 19.64,72.41 POTI-SCHALTER-BOX.2 | 60.96,59.69 66.04,59.69 ESP32-2-RIGHT2.4 ESP32-2-RIGHT1.4 60.96,59.69
  other vias: 50.8,69.85 48.26,67.31 45.72,67.31 43.18,67.31 40.64,67.31 60.96,90.17 71.12,87.63 73.66,87.63 83.82,87.63 86.36,90.17 88.9,87.63 91.44,87.63 99.06,97.79 96.52,95.25 106.68,90.17 99.06,82.55 129.54,77.47 134.62,82.55 134.62,90.17 139.7,85.09 144.78,77.47 154.94,87.63 157.48,49.53 147.32,39.37 144.78,31.75 124.46,13.97 114.3,19.05 111.76,5.08 101.6,10.16 99.06,13.97 88.9,10.16 86.36,16.51 78.74,16.51 83.82,24.13 71.12,21.59 63.5,19.05 58.42,19.05 53.34,21.59 46.99,12.7 43.18,13.97 43.18,16.51 40.64,16.51 38.1,16.51 35.56,19.05 30.48,19.05 38.1,24.13 40.64,24.13 45.72,26.67 38.1,34.29 45.72,41.91 35.56,46.99 50.8,59.69 68.58,52.07 68.58,57.15 68.58,49.53 68.58,46.99 68.58,67.31 71.12,67.31 73.66,67.31 83.82,67.31 111.76,72.39 132.08,64.77 129.54,52.07 132.08,49.53 132.08,46.99 124.46,46.99 119.38,49.53 114.3,46.99 68.58,36.83 68.58,34.29 73.66,34.29
N$ESP2-IO16  (4 unrouted)
  Top 0.813: 68.58,49.53 86.36,49.53 99.06,36.83 99.06,13.97
  Bottom 0.813: ESP32-2-RIGHT1.8 ESP32-2-RIGHT2.8 68.58,49.53 | 99.06,13.97 IO17.1
N$ESP2-IO17  (4 unrouted)
  Top 0.813: 68.58,46.99 81.28,46.99 86.36,41.91 86.36,16.51
  Bottom 0.813: 68.58,46.99 ESP32-2-RIGHT2.9 ESP32-2-RIGHT1.9 | 86.36,16.51 IO16.1
N$ESP2-IO18  (via drill 0.76)  (4 unrouted)
  Top 0.813: 45.72,87.65 v45.72,87.63 45.72,67.33
  Bottom 0.813: SD-BOX.7 45.72,87.65 | 45.72,67.33 45.72,47.01 50.8,41.93 ESP32-2-RIGHT1.11 ESP32-2-RIGHT2.11
N$ESP2-IO19  (via drill 0.76)  (4 unrouted)
  Top 0.813: 40.64,87.65 v40.64,87.63 40.64,67.33
  Bottom 0.813: SD-BOX.5 40.64,87.65 | 40.64,67.33 40.64,44.47 45.72,39.39 ESP32-2-RIGHT1.12 ESP32-2-RIGHT2.12
N$ESP2-IO21  (6 unrouted)
  Top 0.813: 71.12,67.33 71.12,87.65 | 68.58,34.31 73.66,34.31
  Bottom 0.813: ESP32-2-RIGHT1.14 ESP32-2-RIGHT2.14 68.58,34.31 | OLED-BOX.4 66.04,92.73 71.12,87.65 | 71.12,67.33 73.66,64.79 73.66,34.31
N$ESP2-IO22  (2 unrouted)
  Top 0.813: 60.96,90.19 68.58,82.57 68.58,67.33
  Bottom 0.813: ESP32-2-RIGHT1.17 ESP32-2-RIGHT2.17 66.06,26.67 68.58,26.67 71.12,29.21 71.12,64.79 68.58,67.33 | OLED-BOX.3 60.96,90.19
N$ESP2-IO23  (via drill 0.76)  (8 unrouted)
  Top 0.813: 43.18,87.65 v43.18,87.63 43.18,67.33 | 45.72,41.93 45.72,26.69
  Bottom 0.813: SD-BOX.6 43.18,87.65 | 43.18,67.33 43.18,44.47 45.72,41.93 | 45.72,26.69 48.26,24.15 ESP32-2-RIGHT1.18 ESP32-2-RIGHT2.18
N$ESP2-IO26  (4 unrouted)
  Top 0.813: 38.1,34.31 43.18,29.23 43.18,16.53 | 111.76,5.1 109.22,2.56 81.28,2.56 76.2,7.64 76.18,7.62 52.07,7.62 46.99,12.7
  Bottom 0.813: 38.1,34.31 38.1,41.93 35.56,44.47 ESP32-2-LEFT1.10 ESP32-2-LEFT2.10 | 111.76,5.1 ENDSCHALTER-REINIGUNG.1 | 43.18,16.53 43.18,16.51 46.99,12.7
N$ESP2-IO32
  Bottom 0.813: R3.1 R1.2 ESP32-2-LEFT2.7 ESP32-2-LEFT1.7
